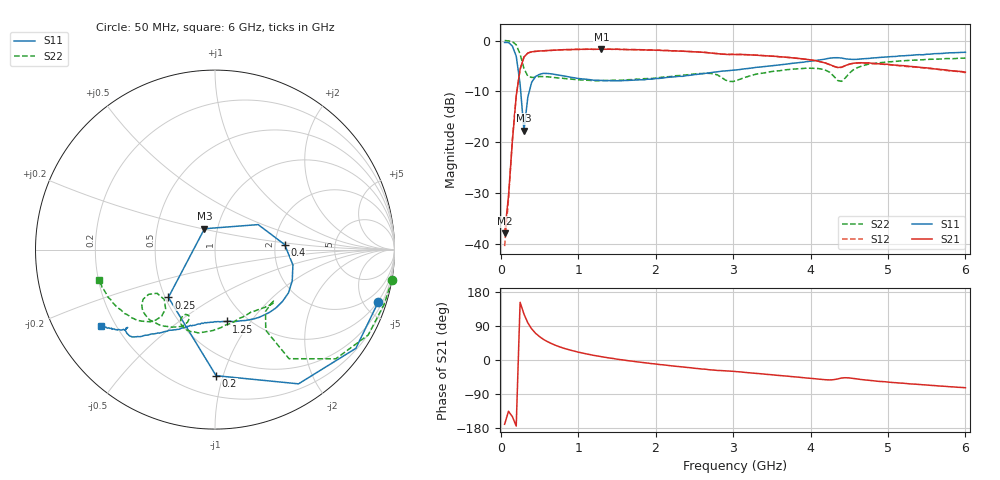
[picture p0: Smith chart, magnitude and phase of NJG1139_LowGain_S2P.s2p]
! Created Fri Jun 05 18:49:35 2009
# hz S ma R 50
! 2 Port Network Data from SP6.SP block
! freq  magS11  angS11  magS21  angS21  magS12  angS12  magS22  angS22
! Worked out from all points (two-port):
!   120 points, 50 MHz to 6 GHz, reference 50 ohm
!   highest |S21| = -1.69 dB at 1.3 GHz (marker M1); lowest = -37.9 dB at 50 MHz (marker M2)
!   |S21| within 3 dB of the highest: 270.1 MHz to 4.24 GHz (3.97 GHz wide, 176 % of centre); 4.494 GHz to 5.005 GHz (511.4 MHz wide, 10.8 % of centre)
!   lowest |S11| = -17.7 dB at 300 MHz (marker M3), VSWR 1.30, Z = 43.3 + j10.2 ohm
!   |S11| at or under -10 dB: 257.7 MHz to 369.2 MHz (111.4 MHz wide, 35.6 % of centre)
!   |S22| runs from -8.1 to 0.0 dB; largest |S21 - S12| = 0.019
!   S11 on the Smith chart (normalised r, x): 50 MHz: 0.94, -6.27; 200 MHz: 0.34, -0.95; 250 MHz: 0.52, -0.32; 400 MHz: 2.26, +0.15; 1.25 GHz: 0.81, -0.77; 6 GHz: 0.14, -0.30
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5e7  0.9554 -17.7  0.01271 -169.6  0.009477 -54.2  1.001 -9.7
1e8  0.9585 -35.0  0.02935 -135.4  0.02734 -125.2  0.9901 -18.1
1.5e8  0.8808 -58.1  0.1015 -149.2  0.1051 -148.1  0.9771 -29.1
2e8  0.7025 -89.5  0.2851 -174.3  0.2858 -174.1  0.9074 -42.1
2.5e8  0.3721 -134.3  0.5217 152.3  0.5208 151.7  0.7346 -55.9
3e8  0.1301 116.8  0.6881 121.3  0.6855 121.0  0.5304 -57.8
3.5e8  0.2779 30.1  0.7529 97.9  0.7527 97.8  0.4447 -50.7
4e8  0.3891 4.1  0.7745 82.0  0.7747 81.8  0.4334 -43.6
5e8  0.4644 -22.1  0.7891 61.9  0.7858 61.6  0.4426 -41.3
6.5e8  0.47 -43.7  0.8009 43.8  0.7981 43.7  0.436 -45.0
1.05e9  0.419 -71.9  0.8195 18.6  0.818 18.5  0.4088 -56.3
1.25e9  0.4056 -80.8  0.8198 10.6  0.8211 10.5  0.4024 -61.7
1.3e9  0.4047 -82.4  0.8236 8.7  0.8214 8.6  0.4034 -63.0
2.05e9  0.424 -102.5  0.801 -12.0  0.8028 -12.1  0.4323 -84.6
2.8e9  0.4924 -115.5  0.7423 -27.6  0.7423 -27.6  0.4582 -114.3
3.05e9  0.5144 -119.2  0.728 -30.8  0.7284 -30.8  0.4052 -110.6
4.05e9  0.6335 -130.3  0.6363 -49.3  0.6348 -49.5  0.532 -136.8
4.35e9  0.6772 -136.5  0.5426 -50.1  0.5418 -50.4  0.4043 -143.0
4.45e9  0.6602 -138.5  0.5664 -46.8  0.5643 -46.9  0.4288 -129.9
4.6e9  0.653 -138.3  0.6018 -49.9  0.5988 -50.3  0.5386 -131.7
5.05e9  0.6947 -140.0  0.5758 -59.2  0.5737 -59.2  0.6191 -145.9
6e9  0.7657 -146.1  0.4883 -73.2  0.4825 -73.0  0.671 -165.2
